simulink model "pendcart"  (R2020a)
settings: Solver=VariableStepAuto  StartTime=0.0  StopTime=10.0  RelTol=1e-3
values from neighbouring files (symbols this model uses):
  g = 9.8    [init_params_FS.m]
  K = [-3.1623 -4.8648 -45.9014 -14.6871]    [init_params_FS.m]
  l = 1    [init_params_FS.m]
  m = 0.1    [init_params_FS.m]
  M = 1    [init_params_FS.m]
  theta0 = 0.55    [init_params_FS.m]
  x0 = 0.2    [init_params_FS.m]

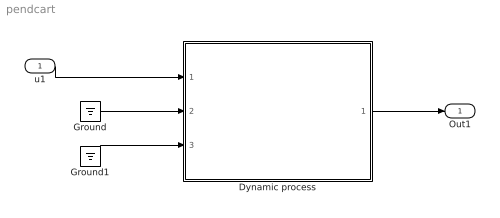
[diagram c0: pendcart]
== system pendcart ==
  u1 : Inport
  Dynamic process : Subsystem
  Ground : Ground
  Ground1 : Ground
  Out1 : Outport
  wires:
  u1/1 -> Dynamic process/1(u1)
  Ground/1 -> Dynamic process/2(u2)
  Ground1/1 -> Dynamic process/3(fs)
  Dynamic process/1(y) -> Out1/1

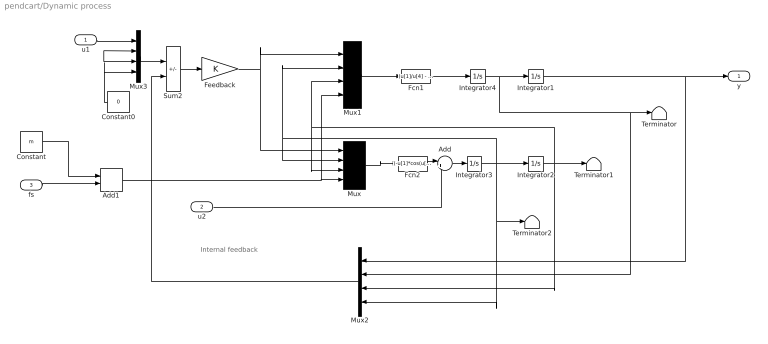
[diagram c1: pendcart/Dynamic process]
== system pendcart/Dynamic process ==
  note: Internal feedback
  u1 : Inport
  u2 : Inport  Port=2
  fs : Inport  Port=3
  Add : Sum  Inputs=|++  InputSameDT=on
  Add1 : Sum
  Constant : Constant  Value=m
  Constant0 : Constant  Value=0
  Fcn1 : Fcn  Expr=(u[1]/u[4] - g*sin(u[3])*cos(u[3]) + l*power(u[2],2)*sin(u[3]))/(M/u[4] + power(sin(u[3]),2))
  Fcn2 : Fcn  Expr=(-u[1]*cos(u[3])/u[4] + (M+u[4])*g*sin(u[3])/u[4] - l*power(u[2],2)*sin(u[3])*cos(u[3]))/(l*(M/u[4] + power(sin(u[3]),2)))
  Feedback : Gain  Gain=K  Multiplication=Matrix(K*u)
  Integrator1 : Integrator  InitialCondition=x0
  Integrator2 : Integrator  InitialCondition=theta0
  Integrator3 : Integrator
  Integrator4 : Integrator
  Mux{,1..3} (4 alike) : Mux
  Sum2 : Sum  Inputs=+-  InputSameDT=on  SaturateOnIntegerOverflow=on
  Terminator : Terminator
  Terminator1 : Terminator
  Terminator2 : Terminator
  y : Outport
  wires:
  Mux/1 -> Fcn2/1
  Mux1/1 -> Fcn1/1
  Fcn1/1 -> Integrator4/1
  Integrator4/1 -> Integrator1/1, Mux2/2, Terminator/1
  Feedback/1 -> Mux/1, Mux1/1
  Integrator3/1 -> Mux1/2, Mux/2, Integrator2/1, Mux2/4, Terminator2/1
  Integrator2/1 -> Mux1/3, Mux/3, Mux2/3, Terminator1/1
  Add/1 -> Integrator3/1
  Fcn2/1 -> Add/1
  Integrator1/1 -> y/1, Mux2/1
  u2/1 -> Add/2
  Sum2/1 -> Feedback/1
  Constant0/1 -> Mux3/2, Mux3/3, Mux3/4
  Mux3/1 -> Sum2/1
  u1/1 -> Mux3/1
  Mux2/1 -> Sum2/2
  Add1/1 -> Mux1/4, Mux/4
  Constant/1 -> Add1/1
  fs/1 -> Add1/2
